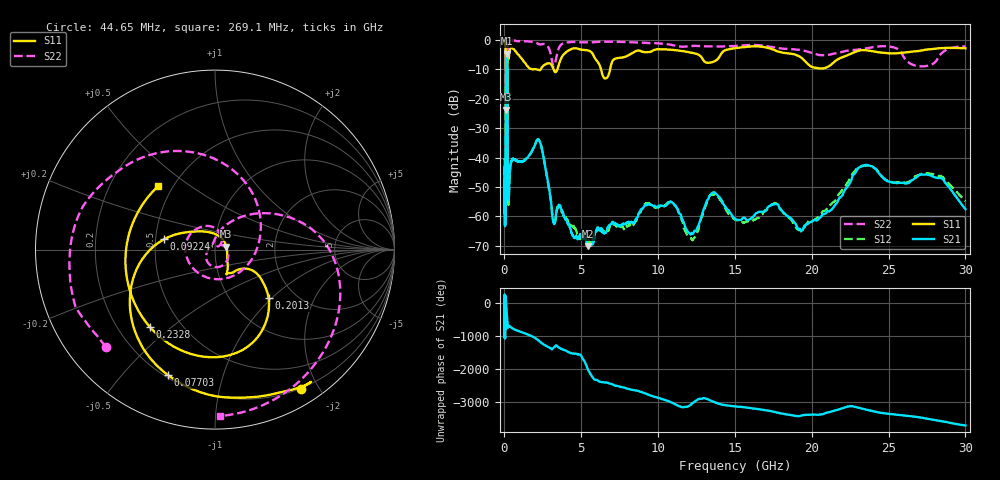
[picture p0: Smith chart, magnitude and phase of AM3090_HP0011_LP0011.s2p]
! Date/Time: Thu, Feb 28, 2019 1:56 PM
! Network Analyzer: Agilent Technologies E8364B Rev: A.07.50.67
! Sweep from 0.010 to 30.000 GHz, 1601 Points, Sweep Type: LOG
! Power Supply: 5.023 V, 0.002 A
# Hz S DB R 50
!freq MagS11 AngS11 MagS21 AngS21 MagS12 AngS12 MagS22 AngS22
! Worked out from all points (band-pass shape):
!   1601 points, 10 MHz to 30 GHz, reference 50 ohm
!   highest |S21| = -4.61 dB at 141.8 MHz (marker M1); lowest = -70.2 dB at 5.419 GHz (marker M2)
!   |S21| within 3 dB of the highest: 101.6 MHz to 188.2 MHz (86.58 MHz wide, 59.7 % of centre)
!   lowest |S11| = -23.7 dB at 100.4 MHz (marker M3), VSWR 1.14, Z = 56.7 + j1.94 ohm
!   |S11| at or under -10 dB: 2.136 GHz to 2.36 GHz (224.3 MHz wide, 9.98 % of centre); 3.199 GHz to 3.446 GHz (246.4 MHz wide, 7.42 % of centre); 6.288 GHz to 6.876 GHz (588 MHz wide, 8.93 % of centre)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
!   |S22| runs from -33.0 to -0.2 dB; largest |S21 - S12| = 0.013
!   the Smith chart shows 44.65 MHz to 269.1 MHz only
!   S11 on the Smith chart (normalised r, x): 44.65 MHz: 0.19, -1.77; 77.03 MHz: 0.21, -0.67; 92.24 MHz: 0.55, +0.07; 201.3 MHz: 1.48, -0.96; 232.8 MHz: 0.33, -0.42; 269.1 MHz: 0.42, +0.38
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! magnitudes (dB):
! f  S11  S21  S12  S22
! 10 MHz  -0.3  -45.6  -40.2  -0.5
! 38.04 MHz  -0.5  -62.8  -60.5  -1.4
! 44.65 MHz  -0.8  -57.2  -58.9  -1.8
! 77.03 MHz  -2.5  -46.4  -46.8  -4.9
! 92.24 MHz  -10.8  -15.4  -15.5  -15.6
! 100.4 MHz  -23.7  -8.1  -8.1  -15.7
! 127.7 MHz  -16.4  -4.8  -4.8  -32.9
! 141.8 MHz  -16.2  -4.6  -4.6  -23.9
! 144.7 MHz  -16.1  -4.6  -4.6  -22.5
! 179.4 MHz  -14.3  -6.2  -6.1  -31.0
! 201.3 MHz  -7.9  -14.5  -14.5  -11.3
! 232.8 MHz  -5.0  -53.2  -54.6  -1.5
! 269.1 MHz  -6.5  -54.2  -56.1  -0.6
! 550.5 MHz  -2.9  -40.5  -40.5  -0.2
! 2.084 GHz  -10.0  -34.4  -34.4  -1.0
! 3.188 GHz  -9.8  -62.1  -61.4  -8.8
! 5.419 GHz  -3.5  -70.2  -69.3  -0.8
! 7.926 GHz  -5.6  -62.3  -63.0  -0.7
! 13.68 GHz  -7.2  -51.8  -52.5  -2.2
! 19.61 GHz  -7.5  -63.0  -63.0  -3.8
! 23.59 GHz  -3.5  -42.5  -42.6  -2.8
! 30 GHz  -2.8  -57.6  -54.9  -2.2
